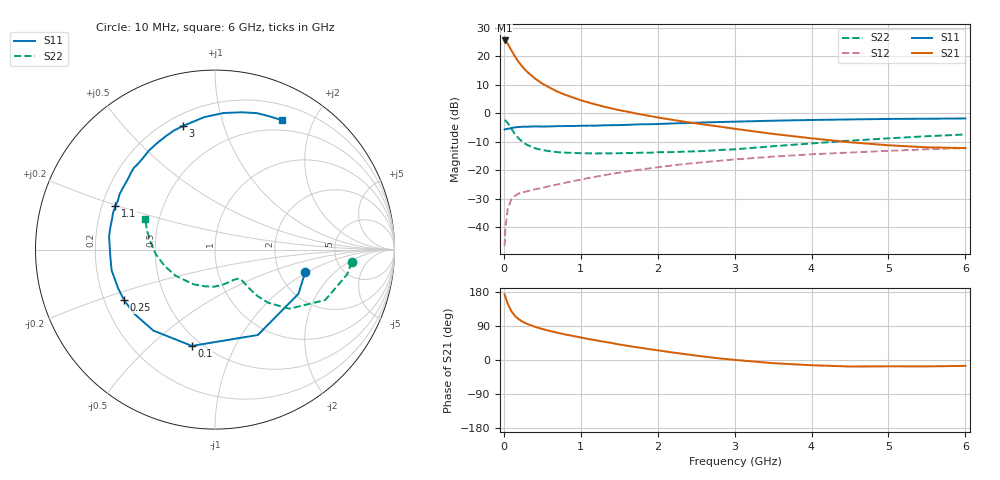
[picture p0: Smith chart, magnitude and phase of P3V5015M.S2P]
! SIEMENS Small Signal Semiconductors
! BFP181
! Si NPN RF Bipolar Junction Transistor in SOT143
! VCE = 0.5 V  IC = 15 mA
! Common Emitter S-Parameters:  March  1996
# GHz  S  MA  R  50
!  f  S11  S21  S12  S22
! GHz  MAG  ANG  MAG  ANG  MAG  ANG  MAG  ANG
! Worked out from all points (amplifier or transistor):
!   36 points, 10 MHz to 6 GHz, reference 50 ohm
!   highest |S21| = 25.6 dB at 10 MHz (marker M1)
!   |S21| within 3 dB of that: start of sweep to 88.64 MHz
!   unconditionally stable (mu >= 1): start of sweep to 18.81 MHz; 216.9 MHz to end of sweep
!   at 250 MHz: K = 1.12, MAG = 19.8 dB, |S12| = -27.8 dB
!   at 1.4 GHz: K = 2.78, MAG = 4.2 dB, |S12| = -21.3 dB
!   at 6 GHz: K = 2.62, MAG = -7.0 dB, |S12| = -12.3 dB
!   S11 on the Smith chart (normalised r, x): 10 MHz: 2.78, -0.96; 100 MHz: 0.45, -0.69; 250 MHz: 0.28, -0.24; 1.1 GHz: 0.25, +0.20; 3 GHz: 0.26, +0.74; 6 GHz: 0.37, +1.57
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0.01  0.5178 -14.1  19.09 173.4  0.0046 74.8  0.7652 -5.2
0.02  0.5262 -27.9  18.8 167.0  0.0092 73.3  0.7493 -10.6
0.05  0.5323 -63.4  16.82 148.8  0.0208 62.8  0.6753 -24.6
0.1  0.5517 -103.5  12.67 128.0  0.0312 46.2  0.5291 -38.5
0.15  0.5672 -127.3  9.721 115.0  0.0358 39.1  0.4201 -44.9
0.2  0.5743 -141.3  7.772 106.6  0.0392 35.4  0.353 -47.5
0.25  0.5799 -150.9  6.386 100.3  0.0408 34.2  0.3096 -48.3
0.3  0.5811 -158.3  5.416 95.5  0.0424 34.0  0.2791 -48.5
0.4  0.5875 -168.6  4.137 87.9  0.0457 34.9  0.2438 -48.8
0.5  0.5844 -176.0  3.328 81.9  0.0488 36.5  0.2256 -49.0
0.6  0.5874 177.9  2.802 76.6  0.0526 38.3  0.2148 -50.1
0.7  0.5943 173.1  2.394 71.9  0.0561 40.1  0.2069 -51.7
0.9  0.5974 164.4  1.89 63.4  0.0644 42.4  0.2009 -56.0
1.1  0.6066 156.5  1.548 55.3  0.0726 44.1  0.1978 -61.2
1.5  0.62 143.9  1.135 41.0  0.0901 44.6  0.1981 -73.0
1.9  0.6422 132.0  0.895 28.4  0.1079 43.1  0.2024 -86.6
2.2  0.6633 123.7  0.764 19.6  0.1215 41.3  0.2078 -98.7
3  0.7122 104.4  0.534 0.3  0.1542 34.8  0.2324 -128.9
3.5  0.7405 94.6  0.434 -8.4  0.173 30.2  0.2632 -146.3
4.5  0.7792 79.0  0.309 -17.2  0.2042 20.1  0.3298 -175.2
5.5  0.8022 67.7  0.252 -16.9  0.2326 11.0  0.395 164.1
6  0.8111 62.8  0.244 -15.5  0.2437 6.1  0.424 156.1
